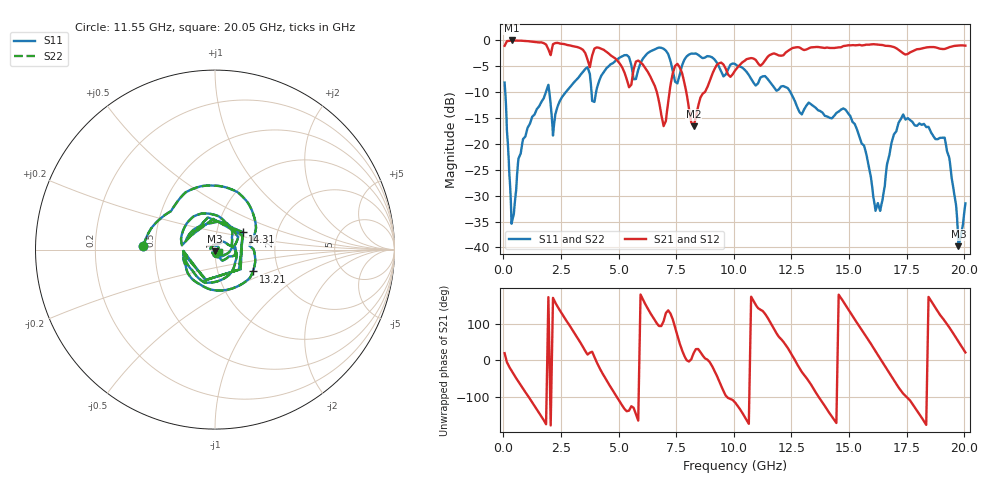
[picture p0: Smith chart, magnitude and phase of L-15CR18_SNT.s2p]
#	mhz	s	ma	r	50
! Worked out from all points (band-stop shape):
!   1001 points, 50 MHz to 20.05 GHz, reference 50 ohm
!   highest |S21| = -0.03 dB at 350 MHz (marker M1); lowest = -16.6 dB at 8.25 GHz (marker M2)
!   |S21| within 3 dB of the highest: start of sweep to 3.596 GHz; 11.51 GHz to end of sweep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
!   lowest |S11| = -39.8 dB at 19.75 GHz (marker M3), VSWR 1.02, Z = 49.9 - j1.03 ohm
!   |S11| at or under -10 dB: 78.53 MHz to 1.842 GHz (1.764 GHz wide, 184 % of centre); 1.992 GHz to 2.707 GHz (714.7 MHz wide, 30.4 % of centre); 12.45 GHz to end of sweep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
!   |S22| runs from -39.8 to -1.4 dB; largest |S21 - S12| = 0
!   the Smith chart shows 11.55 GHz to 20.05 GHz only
!   S11 on the Smith chart (normalised r, x): 11.55 GHz: 0.43, +0.02; 13.21 GHz: 1.48, -0.38; 14.31 GHz: 1.33, +0.27; 20.05 GHz: 1.05, -0.03
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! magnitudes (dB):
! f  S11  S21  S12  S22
! 50 MHz  -8.2  -1.1  -1.1  -8.2
! 350 MHz  -35.4  0.0  0.0  -35.4
! 1.87 GHz  -9.6  -1.0  -1.0  -9.6
! 2.19 GHz  -16.5  -0.7  -0.7  -16.5
! 3.39 GHz  -6.4  -1.7  -1.7  -6.4
! 3.93 GHz  -11.9  -1.8  -1.8  -11.9
! 6.73 GHz  -1.4  -11.4  -11.4  -1.4
! 6.99 GHz  -1.8  -16.2  -16.2  -1.8
! 7.57 GHz  -8.0  -4.7  -4.7  -8.0
! 8.25 GHz  -2.6  -16.6  -16.6  -2.6
! 10.05 GHz  -4.6  -5.8  -5.8  -4.6
! 11.55 GHz  -8.0  -2.9  -2.9  -8.0
! 13.21 GHz  -12.3  -1.6  -1.6  -12.3
! 13.39 GHz  -12.5  -1.4  -1.4  -12.5
! 14.31 GHz  -14.8  -1.5  -1.5  -14.8
! 15.29 GHz  -16.6  -1.0  -1.0  -16.6
! 16.23 GHz  -31.7  -0.8  -0.8  -31.7
! 16.73 GHz  -22.5  -1.1  -1.1  -22.5
! 17.33 GHz  -14.5  -2.5  -2.5  -14.5
! 19.09 GHz  -18.8  -1.7  -1.7  -18.8
! 19.75 GHz  -39.8  -1.0  -1.0  -39.8
! 20.05 GHz  -31.5  -1.0  -1.0  -31.5
